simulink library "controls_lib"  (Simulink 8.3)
settings: Solver=ode45  StartTime=0.0  StopTime=10.0  RelTol=1e-3
undefined symbols (not defined in the file or in its folder): controls
libraries: general_lib x5, simulink x2

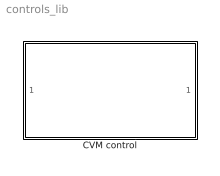
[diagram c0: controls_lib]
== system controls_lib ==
  CVM control : Subsystem

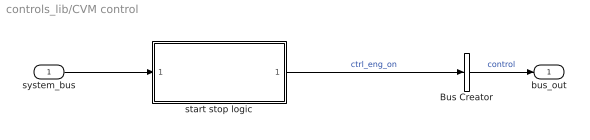
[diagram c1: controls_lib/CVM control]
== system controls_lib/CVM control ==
  system_bus : Inport
  Bus Creator : BusCreator  Inputs=1
  start stop logic : Subsystem
  bus_out : Outport
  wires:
  Bus Creator/1 -> bus_out/1  "control"
  system_bus/1 -> start stop logic/1(system_bus)
  start stop logic/1(engine_on) -> Bus Creator/1  "ctrl_eng_on"

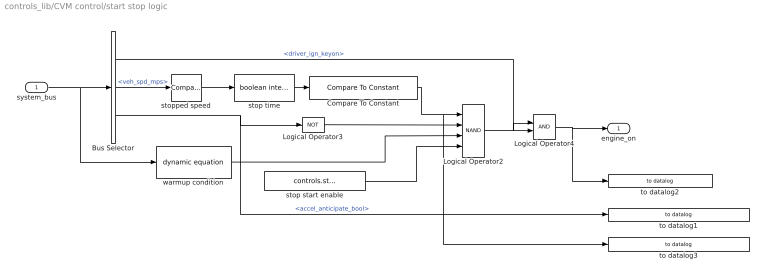
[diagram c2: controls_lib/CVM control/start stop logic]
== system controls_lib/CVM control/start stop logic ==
  system_bus : Inport
  Bus Selector : BusSelector  OutputSignals=driver.driver_ign_keyon,vehicle.veh_spd_mps,driver.accel_anticipate_bool
  Compare To Constant : simulink/Logic and Bit Operations/Compare To Constant  relop=>=  const=controls.stop_delay_secs  OutDataTypeStr=boolean
  Logical Operator2 : Logic  Operator=NAND  Inputs=4  AllPortsSameDT=off  OutDataTypeStr=boolean
  Logical Operator3 : Logic  Operator=NOT  AllPortsSameDT=off  OutDataTypeStr=boolean
  Logical Operator4 : Logic  AllPortsSameDT=off  OutDataTypeStr=boolean
  stop start enable : Constant  Value=controls.start_stop_enable
  stop time : general_lib/boolean integrator  UpperSaturationLimit=Inf  Normalize=off
  stopped speed : simulink/Logic and Bit Operations/Compare To Constant  relop=<=  const=0.1  OutDataTypeStr=boolean
  to datalog1 : general_lib/to datalog  VarName=controls.accel_anticipate_bool  WorkspaceName=datalog__controls__accel_anticipate_bool  VerboseLevel=1  VerboseSignal=REVS.verbose
  to datalog2 : general_lib/to datalog  VarName=controls.engine_on  WorkspaceName=datalog__controls__engine_on  VerboseLevel=1  VerboseSignal=REVS.verbose
  to datalog3 : general_lib/to datalog  VarName=controls.vehicle_stopped_bool  WorkspaceName=datalog__controls__vehicle_stopped_bool  VerboseLevel=1  VerboseSignal=REVS.verbose
  warmup condition : general_lib/dynamic equation  DynamicExpression=controls.start_stop_warmup_condition  DynamicExpressionEval=@cycle_pos_secs > 100
  engine_on : Outport
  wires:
  Logical Operator4/1 -> engine_on/1, to datalog2/1
  Logical Operator2/1 -> Logical Operator4/2
  Compare To Constant/1 -> Logical Operator2/1, to datalog3/1
  Bus Selector/2 -> stopped speed/1  "<veh_spd_mps>"
  Logical Operator3/1 -> Logical Operator2/2
  stop start enable/1 -> Logical Operator2/4
  Bus Selector/3 -> to datalog1/1, Logical Operator3/1  "<accel_anticipate_bool>"
  warmup condition/1 -> Logical Operator2/3
  system_bus/1 -> warmup condition/1, Bus Selector/1
  stopped speed/1 -> stop time/1
  stop time/1 -> Compare To Constant/1
  Bus Selector/1 -> Logical Operator4/1  "<driver_ign_keyon>"
